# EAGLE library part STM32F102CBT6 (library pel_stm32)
STM32F103 Medium Density 48pins
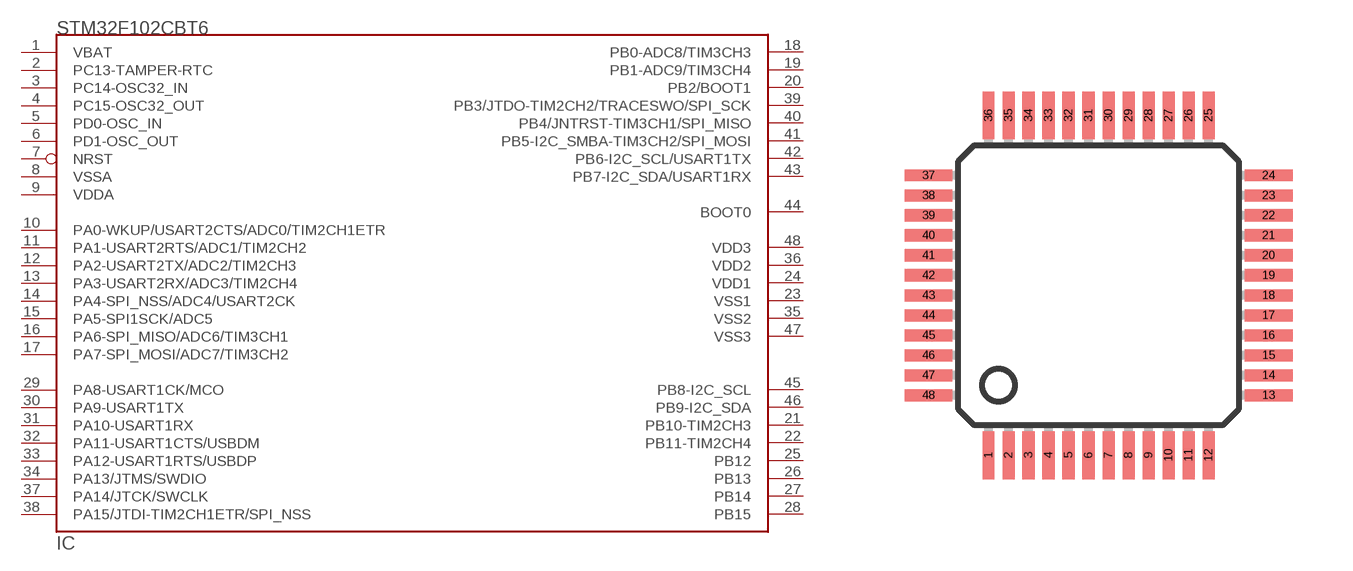
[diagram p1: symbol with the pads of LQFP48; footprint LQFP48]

Designator prefix IC

## STM32F102CBT6  [LQFP48]
1  VBAT  sup
2  PC13-TAMPER-RTC
3  PC14-OSC32_IN
4  PC15-OSC32_OUT
5  PD0-OSC_IN  in
6  PD1-OSC_OUT  out
7  NRST
8  VSSA  sup
9  VDDA  sup
10  PA0-WKUP/USART2CTS/ADC0/TIM2CH1ETR
11  PA1-USART2RTS/ADC1/TIM2CH2
12  PA2-USART2TX/ADC2/TIM2CH3
13  PA3-USART2RX/ADC3/TIM2CH4
14  PA4-SPI_NSS/ADC4/USART2CK
15  PA5-SPI1SCK/ADC5
16  PA6-SPI_MISO/ADC6/TIM3CH1
17  PA7-SPI_MOSI/ADC7/TIM3CH2
18  PB0-ADC8/TIM3CH3
19  PB1-ADC9/TIM3CH4
20  PB2/BOOT1
21  PB10-TIM2CH3
22  PB11-TIM2CH4
23  VSS1  sup
24  VDD1  sup
25  PB12
26  PB13
27  PB14
28  PB15
29  PA8-USART1CK/MCO
30  PA9-USART1TX
31  PA10-USART1RX
32  PA11-USART1CTS/USBDM
33  PA12-USART1RTS/USBDP
34  PA13/JTMS/SWDIO
35  VSS2  sup
36  VDD2  sup
37  PA14/JTCK/SWCLK
38  PA15/JTDI-TIM2CH1ETR/SPI_NSS
39  PB3/JTDO-TIM2CH2/TRACESWO/SPI_SCK
40  PB4/JNTRST-TIM3CH1/SPI_MISO
41  PB5-I2C_SMBA-TIM3CH2/SPI_MOSI
42  PB6-I2C_SCL/USART1TX
43  PB7-I2C_SDA/USART1RX
44  BOOT0  in
45  PB8-I2C_SCL
46  PB9-I2C_SDA
47  VSS3  sup
48  VDD3  sup

## Footprint LQFP48 (pad centres in mm)
Based on STM PCB layout recomendations.
smd 0.3 x 1.2: 1 -2.75,-4.25; 2 -2.25,-4.25; 3 -1.75,-4.25; 4 -1.25,-4.25; 5 -0.75,-4.25; 6 -0.25,-4.25; 7 0.25,-4.25; 8 0.75,-4.25; 9 1.25,-4.25; 10 1.75,-4.25; 11 2.25,-4.25; 12 2.75,-4.25; 25 2.75,4.25; 26 2.25,4.25; 27 1.75,4.25; 28 1.25,4.25; 29 0.75,4.25; 30 0.25,4.25; 31 -0.25,4.25; 32 -0.75,4.25; 33 -1.25,4.25; 34 -1.75,4.25; 35 -2.25,4.25; 36 -2.75,4.25
smd 1.2 x 0.3: 13 4.25,-2.75; 14 4.25,-2.25; 15 4.25,-1.75; 16 4.25,-1.25; 17 4.25,-0.75; 18 4.25,-0.25; 19 4.25,0.25; 20 4.25,0.75; 21 4.25,1.25; 22 4.25,1.75; 23 4.25,2.25; 24 4.25,2.75; 37 -4.25,2.75; 38 -4.25,2.25; 39 -4.25,1.75; 40 -4.25,1.25; 41 -4.25,0.75; 42 -4.25,0.25; 43 -4.25,-0.25; 44 -4.25,-0.75; 45 -4.25,-1.25; 46 -4.25,-1.75; 47 -4.25,-2.25; 48 -4.25,-2.75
